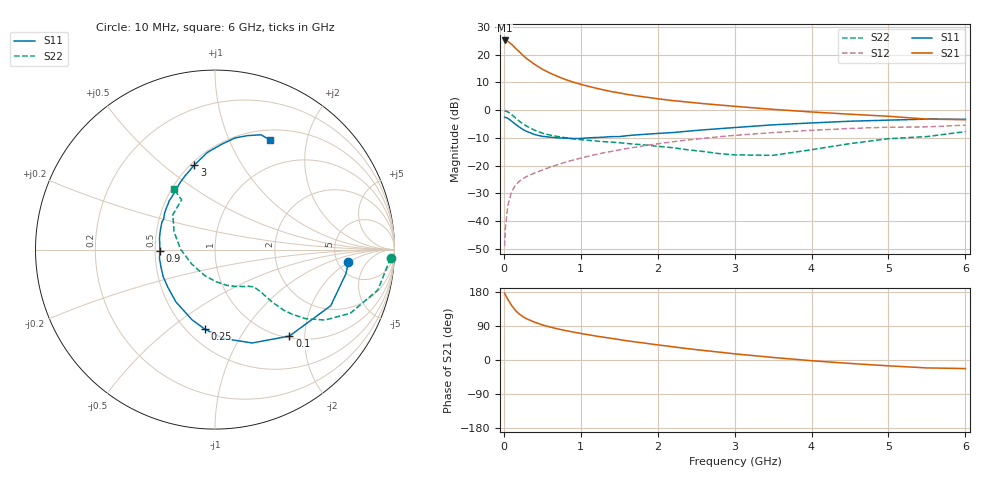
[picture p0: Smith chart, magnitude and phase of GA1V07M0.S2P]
! Infineon Technologies  Discrete & RF Semiconductors
! BF775
! Si NPN RF Bipolar Junction Transistor in SOT23
! VCE = 1 V  IC = 7 mA
! Common Emitter S-Parameters:  May  1996
# GHz  S  MA  R  50
!  f  S11  S21  S12  S22
! GHz  MAG  ANG  MAG  ANG  MAG  ANG  MAG  ANG
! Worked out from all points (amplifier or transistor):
!   36 points, 10 MHz to 6 GHz, reference 50 ohm
!   highest |S21| = 25.2 dB at 10 MHz (marker M1)
!   |S21| within 3 dB of that: start of sweep to 159.2 MHz
!   unconditionally stable (mu >= 1): 588.7 MHz to end of sweep
!   at 250 MHz: K = 0.62, MSG = 22.2 dB, |S12| = -24.7 dB
!   at 1.4 GHz: K = 1.17, MAG = 8.3 dB, |S12| = -14.9 dB
!   at 6 GHz: K = 1.03, MAG = -0.1 dB, |S12| = -5.4 dB
!   S11 on the Smith chart (normalised r, x): 10 MHz: 6.26, -1.99; 100 MHz: 1.04, -1.68; 250 MHz: 0.61, -0.68; 900 MHz: 0.53, -0.01; 3 GHz: 0.52, +0.64; 6 GHz: 0.62, +1.43
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0.01  0.7471 -5.4  18.15 176.2  0.0035 89.1  0.9794 -2.8
0.02  0.7415 -10.5  17.89 172.0  0.0073 85.0  0.9636 -5.7
0.05  0.7165 -25.9  17.49 160.7  0.0185 77.5  0.9351 -13.9
0.1  0.6355 -49.3  15.52 144.3  0.0333 67.1  0.8332 -25.2
0.15  0.56 -68.3  13.21 131.0  0.0441 60.5  0.7283 -32.6
0.2  0.4967 -84.8  11.38 121.4  0.0516 57.1  0.635 -37.3
0.25  0.4469 -97.3  9.732 114.0  0.058 55.3  0.5627 -39.9
0.3  0.4112 -108.2  8.473 108.3  0.0638 54.6  0.511 -41.4
0.4  0.3636 -126.9  6.718 99.7  0.0733 54.7  0.4347 -42.5
0.5  0.3366 -141.1  5.494 92.6  0.0829 55.5  0.3848 -42.7
0.6  0.326 -152.3  4.672 87.1  0.0932 56.3  0.3549 -42.7
0.7  0.3161 -162.2  4.066 82.1  0.1037 56.5  0.3349 -43.0
0.9  0.3077 -178.8  3.218 73.8  0.1257 57.1  0.304 -43.8
1.1  0.3158 168.3  2.694 66.6  0.1475 56.9  0.2854 -46.2
1.3  0.3256 158.1  2.314 60.1  0.1699 55.9  0.2703 -48.9
1.6  0.3458 144.5  1.93 50.7  0.2032 53.5  0.2506 -54.9
2.2  0.3949 123.8  1.487 34.8  0.2692 47.3  0.2098 -71.7
3  0.4854 103.7  1.174 16.3  0.3507 37.1  0.1559 -111.3
3.5  0.5436 94.4  1.034 6.7  0.3941 30.1  0.153 -148.8
4.5  0.6321 79.8  0.845 -9.1  0.4672 16.6  0.249 156.3
5.5  0.689 68.2  0.69 -20.9  0.4988 2.8  0.3338 123.8
6  0.6836 63.3  0.673 -22.6  0.5367 -1.1  0.4096 124.3
